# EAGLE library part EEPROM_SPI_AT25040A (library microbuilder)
AT25010a/40a EEPROM SOIC8 AT25010a, 1K (128 x 8 bit) - Digikey: AT25010AN-10SU2.7-ND AT25040a, 4K (256 x 8 bit) - Digikey: AT25040AN-10SU1.8-ND TSSOP8 AT25010a, 1K (128 x 8 bit) - Digikey: AT25010A-10TU-1.8-ND AT25040a, 4K (256 x 8 bit) - Digikey: AT25040A-10TU-1.8-ND
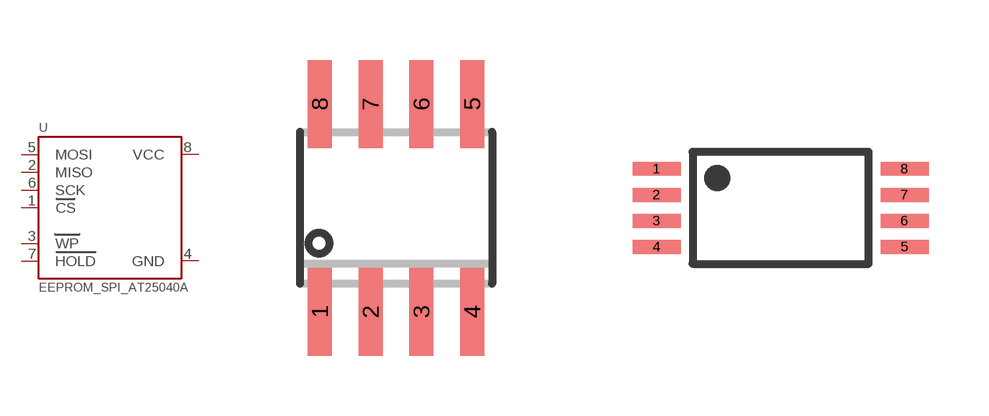
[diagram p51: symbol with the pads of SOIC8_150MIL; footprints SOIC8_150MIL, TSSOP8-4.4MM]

Designator prefix U

## EEPROM_SPI_AT25040A  [SOIC8_150MIL]
1  CS
2  MISO
3  WP
4  GND  pwr
5  MOSI
6  SCK
7  HOLD
8  VCC  pwr

## EEPROM_SPI_AT25040ATSSOP  [TSSOP8-4.4MM]
Pads as for SOIC8_150MIL

## Footprint SOIC8_150MIL (pad centres in mm)
Small Outline IC - 150mil Wide
smd 0.6 x 2.2: 1 -1.905,-2.6; 2 -0.635,-2.6; 3 0.635,-2.6; 4 1.905,-2.6; 5 1.905,2.6; 6 0.635,2.6; 7 -0.635,2.6; 8 -1.905,2.6

## Footprint TSSOP8-4.4MM (pad centres in mm)
Thin Shrink Small Outline Package 0.65mm Pitch, 4.4mm x 3.0mm Body
smd 1.2 x 0.35: 1 -3.1,0.975; 2 -3.1,0.325; 3 -3.1,-0.325; 4 -3.1,-0.975; 5 3.1,-0.975; 6 3.1,-0.325; 7 3.1,0.325; 8 3.1,0.975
